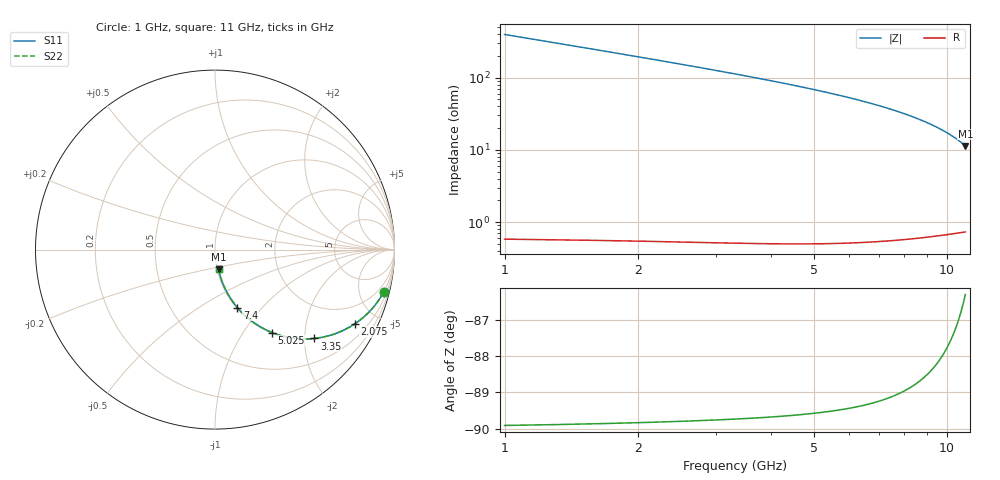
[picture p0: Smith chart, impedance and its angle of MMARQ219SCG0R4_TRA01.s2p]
! MMARQ219SCG0R4_TRA01  S-PARAMETER MODEL  ( General Type )
! Model Generated by TAIYO YUDEN Corporation (http://www.ty-top.com)
! Version 1.0
! TAIYO YUDEN Control No. 210622
! Copyright(c) 2016 TAIYO YUDEN CO.,LTD. All Rights Reserved.
! Product Description (link to TY-COMPAS)
! https://ds.yuden.co.jp/TYCOMPAS/or/detail?pn=MMARQ219SCG0R4ATRA01&u=M
! Products Name : Multilayer Ceramic Capacitors
! Characteristics :
!  Capacitance : 0.4 pF , Rated Voltage : 250V , TCC : CG / C0G
!  Case Size : 2.0 x 1.25 / 0.079 x 0.049 [mm/inch] , Thickness : 0.85 / 0.033 [mm/inch]
!  (Conditions: Temperature = 25 degC , DC Bias Current/Voltage = 0A / 0V)
! External Node Assignments :
!  1  o---| |---o  2
! GND o---------o GND
! Frequency Range : 1000MHz  -  11000MHz  [ 401 STEP ]
# MHZ S RI R 50
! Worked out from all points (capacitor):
!   401 points, 1 GHz to 11 GHz, reference 50 ohm
!   read as one part in series: C = 405 fF near 1.05 GHz
!   lowest |Z| = 11.4 ohm at 11 GHz (marker M1)
!   S11 on the Smith chart (normalised r, x): 1 GHz: 1.01, -7.93; 2.075 GHz: 1.01, -3.75; 3.35 GHz: 1.01, -2.23; 5.025 GHz: 1.01, -1.36; 7.4 GHz: 1.01, -0.74; 11 GHz: 1.01, -0.23
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1000  0.9398 -0.2371  0.0602 0.2371  0.0602 0.2371  0.9398 -0.2371
1275  0.9052 -0.2921  0.0948 0.2921  0.0948 0.2921  0.9052 -0.2921
1500  0.8726 -0.3323  0.1274 0.3323  0.1274 0.3323  0.8726 -0.3323
1775  0.8289 -0.3753  0.1711 0.3753  0.1711 0.3753  0.8289 -0.3753
2075  0.7778 -0.4143  0.2222 0.4143  0.2222 0.4143  0.7778 -0.4143
2375  0.7247 -0.445  0.2753 0.445  0.2753 0.445  0.7247 -0.445
2675  0.6711 -0.468  0.3289 0.468  0.3289 0.468  0.6711 -0.468
3000  0.6137 -0.4849  0.3863 0.4849  0.3863 0.4849  0.6137 -0.4849
3350  0.5539 -0.4948  0.4461 0.4948  0.4461 0.4948  0.5539 -0.4948
3825  0.4778 -0.4969  0.5222 0.4969  0.5222 0.4969  0.4778 -0.4969
4350  0.4019 -0.4872  0.5981 0.4872  0.5981 0.4872  0.4019 -0.4872
5025  0.3176 -0.4619  0.6824 0.4619  0.6824 0.4619  0.3176 -0.4619
5500  0.267 -0.4382  0.733 0.4382  0.733 0.4382  0.267 -0.4382
6000  0.221 -0.4101  0.779 0.4101  0.779 0.4101  0.221 -0.4101
6675  0.1692 -0.3691  0.8308 0.3691  0.8308 0.3691  0.1692 -0.3691
7400  0.125 -0.3234  0.875 0.3234  0.875 0.3234  0.125 -0.3234
7675  0.1108 -0.3059  0.8892 0.3059  0.8892 0.3059  0.1108 -0.3059
8575  0.0732 -0.2497  0.9268 0.2497  0.9268 0.2497  0.0732 -0.2497
9350  0.0496 -0.2029  0.9504 0.2029  0.9504 0.2029  0.0496 -0.2029
10200  0.0312 -0.154  0.9688 0.154  0.9688 0.154  0.0312 -0.154
10550  0.0256 -0.1346  0.9744 0.1346  0.9744 0.1346  0.0256 -0.1346
11000  0.0197 -0.1104  0.9803 0.1104  0.9803 0.1104  0.0197 -0.1104
